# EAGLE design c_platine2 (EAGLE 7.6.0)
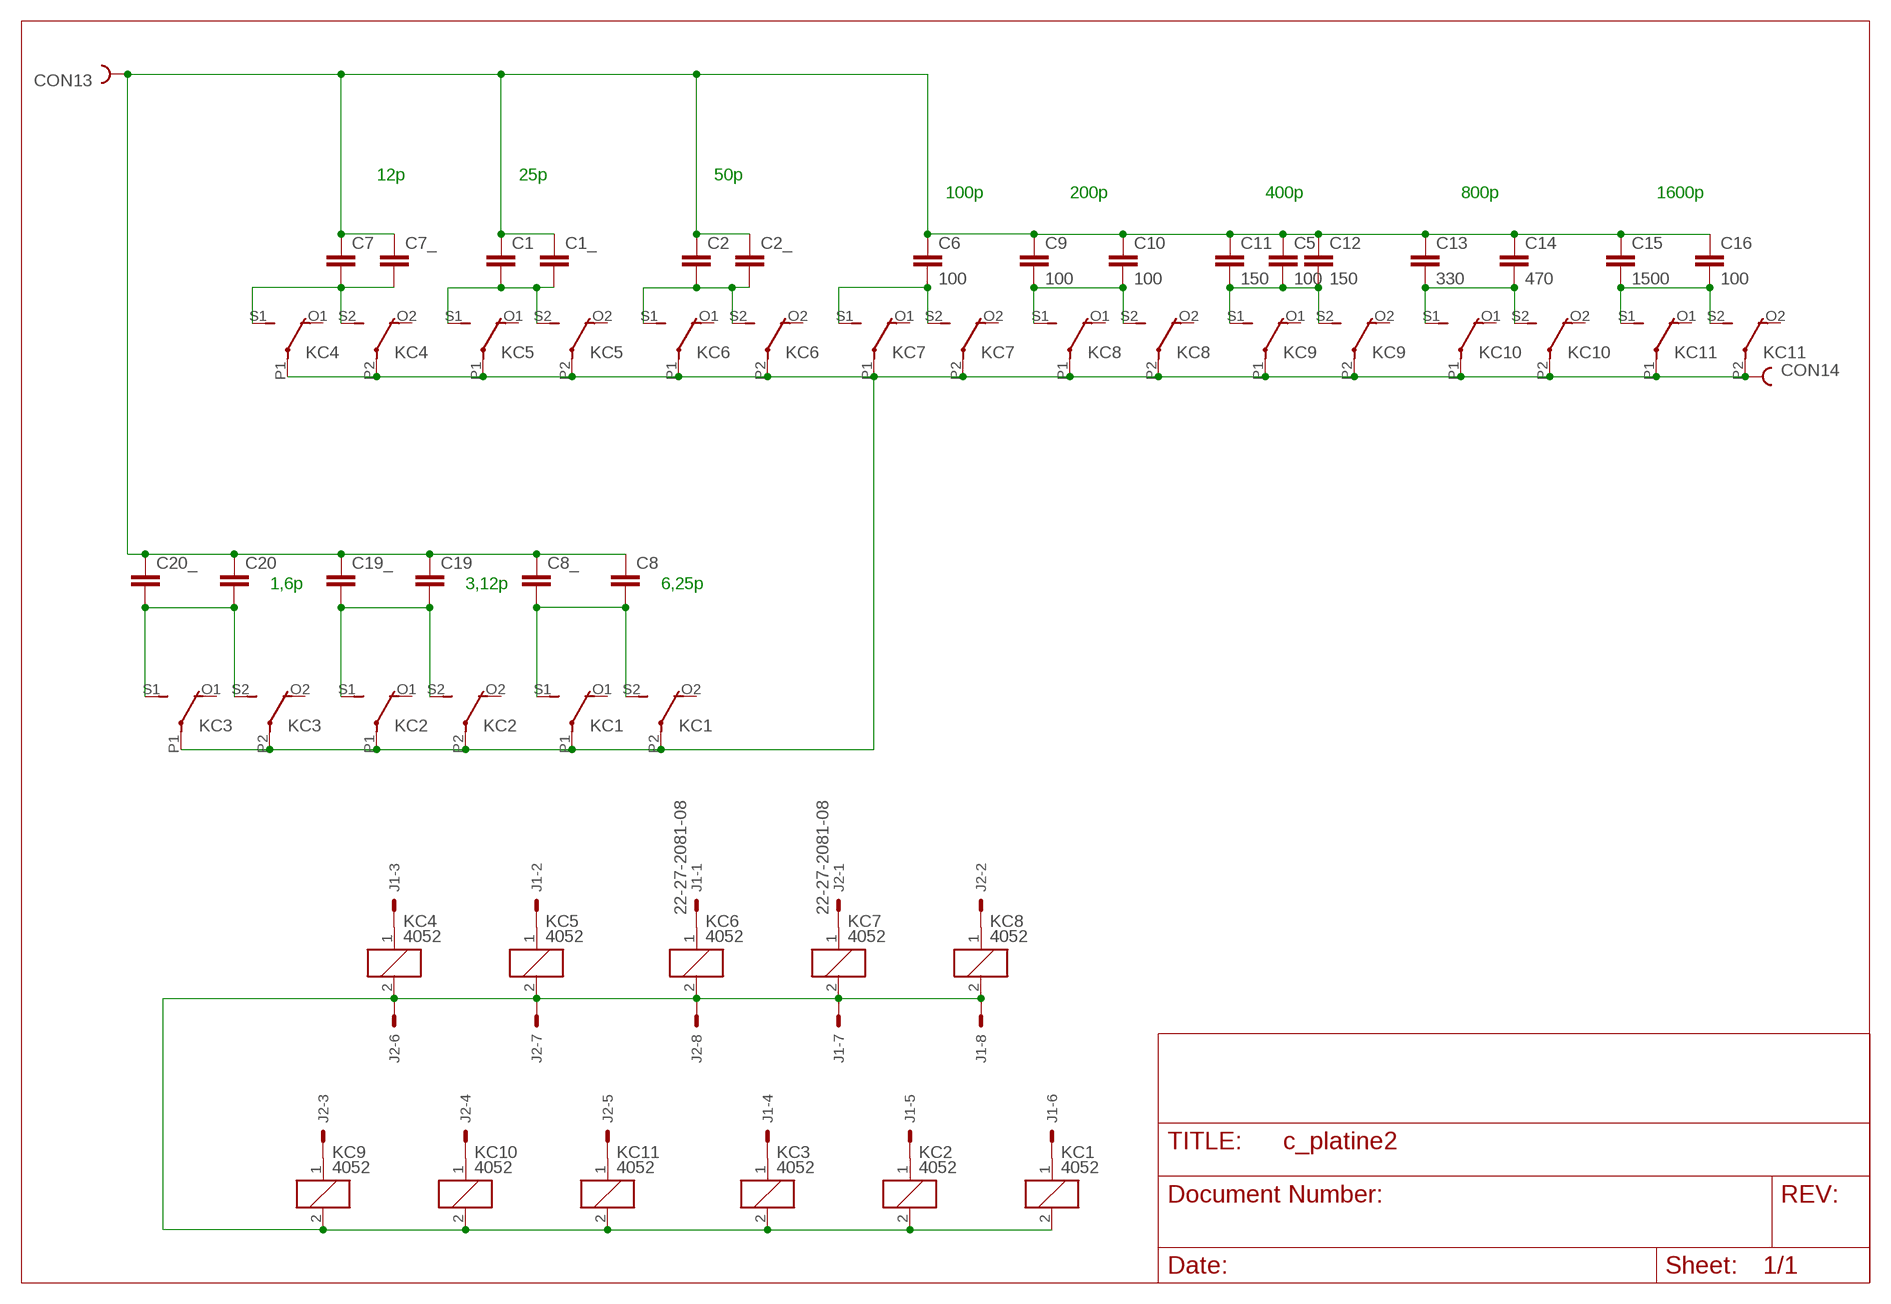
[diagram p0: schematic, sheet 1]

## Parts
C1  C-EUC1812K  [C1812K]
C1_  C-EU102-043X133  [C102-043X133]
C2  C-EUC1812K  [C1812K]
C2_  C-EU102-043X133  [C102-043X133]
C5  100  C-EU150-054X183  [C150-054X183]
C6  100  C-EU150-054X183  [C150-054X183]
C7  C-EUC1812K  [C1812K]
C7_  C-EU102-043X133  [C102-043X133]
C8  C-EUC1812K  [C1812K]
C8_  C-EU102-043X133  [C102-043X133]
C9  100  C-EU150-054X183  [C150-054X183]
C10  100  C-EU150-054X183  [C150-054X183]
C11  150  C-EU150-054X183  [C150-054X183]
C12  150  C-EU150-054X183  [C150-054X183]
C13  330  C-EU150-054X183  [C150-054X183]
C14  470  C-EU150-054X183  [C150-054X183]
C15  1500  C-EU225-074X268  [C225-074X268]
C16  100  C-EU150-054X183  [C150-054X183]
C19  C-EUC1812K  [C1812K]
C19_  C-EU102-043X133  [C102-043X133]
C20  C-EUC1812K  [C1812K]
C20_  C-EU102-043X133  [C102-043X133]
CON13  PIN2_53MM  [HOLE3]
CON14  PIN2_53MM  [HOLE3]
J1  22-27-2081-08  [6410-08]
J2  22-27-2081-08  [6410-08]
KC1  4052  [F4052]
KC2  4052  [F4052]
KC3  4052  [F4052]
KC4  4052  [F4052]
KC5  4052  [F4052]
KC6  4052  [F4052]
KC7  4052  [F4052]
KC8  4052  [F4052]
KC9  4052  [F4052]
KC10  4052  [F4052]
KC11  4052  [F4052]

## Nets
N$1: CON14.1 KC1.P1(2:P) KC1.P2(3:P) KC2.P1(2:P) KC2.P2(3:P) KC3.P1(2:P) KC3.P2(3:P) KC4.P1(2:P) KC4.P2(3:P) KC5.P1(2:P) KC5.P2(3:P) KC6.P1(2:P) KC6.P2(3:P) KC7.P1(2:P) KC7.P2(3:P) KC8.P1(2:P) KC8.P2(3:P) KC9.P1(2:P) KC9.P2(3:P) KC10.P1(2:P) KC10.P2(3:P) KC11.P1(2:P) KC11.P2(3:P)
N$2: C8.2 C8_.2 KC1.S1(2:S) KC1.S2(3:S)
N$3: C1.2 C1_.2 KC5.S1(2:S) KC5.S2(3:S)
N$4: C2.2 C2_.2 KC6.S1(2:S) KC6.S2(3:S)
N$5: C6.2 KC7.S1(2:S) KC7.S2(3:S)
N$6: C7.2 C7_.2 KC4.S1(2:S) KC4.S2(3:S)
N$7: C9.2 C10.2 KC8.S1(2:S) KC8.S2(3:S)
N$8: C5.2 C11.2 C12.2 KC9.S1(2:S) KC9.S2(3:S)
N$9: C13.2 C14.2 KC10.S1(2:S) KC10.S2(3:S)
N$10: C15.2 C16.2 KC11.S1(2:S) KC11.S2(3:S)
N$12: J1.6 KC1.1
N$13: J1.5 KC2.1
N$14: J1.2 KC5.1
N$15: C1.1 C1_.1 C2.1 C2_.1 C5.1 C6.1 C7.1 C7_.1 C8.1 C8_.1 C9.1 C10.1 C11.1 C12.1 C13.1 C14.1 C15.1 C16.1 C19.1 C19_.1 C20.1 C20_.1 CON13.1
N$16: J1.7 J1.8 J2.6 J2.7 J2.8 KC1.2 KC2.2 KC3.2 KC4.2 KC5.2 KC6.2 KC7.2 KC8.2 KC9.2 KC10.2 KC11.2
N$17: J1.1 KC6.1
N$18: C20.2 C20_.2 KC3.S1(2:S) KC3.S2(3:S)
N$19: J2.1 KC7.1
N$20: C19.2 C19_.2 KC2.S1(2:S) KC2.S2(3:S)
N$21: J1.4 KC3.1
N$22: J2.5 KC11.1
N$23: J2.3 KC9.1
N$24: J2.4 KC10.1
N$25: J2.2 KC8.1
N$26: J1.3 KC4.1
Unconnected: KC1.O1(2:O) KC1.O2(3:O) KC2.O1(2:O) KC2.O2(3:O) KC3.O1(2:O) KC3.O2(3:O) KC4.O1(2:O) KC4.O2(3:O) KC5.O1(2:O) KC5.O2(3:O) KC6.O1(2:O) KC6.O2(3:O) KC7.O1(2:O) KC7.O2(3:O) KC8.O1(2:O) KC8.O2(3:O) KC9.O1(2:O) KC9.O2(3:O) KC10.O1(2:O) KC10.O2(3:O) KC11.O1(2:O) KC11.O2(3:O)

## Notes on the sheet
- 12p | 25p | 50p
- 100p | 200p | 400p | 800p | 1600p
- 1,6p | 3,12p | 6,25p

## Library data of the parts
C1 C1_ C2 C2_ C5-C7 C7_ C8 C8_ C9-C16 C19 C19_ C20 C20_ = rcl:C-EU: CAPACITOR, European symbol
CON13 CON14 = lindenau:PIN2_5
J1 J2 = con-molex:22-?-08: CONNECTOR wire to board 2.54 mm (.1 inch) pitch header; OC_FARNELL: unknown; OC_NEWARK: unknown
KC1-KC11 = relay:4052: RELAY 2 x switch, Finder; OC_FARNELL: unknown; OC_NEWARK: unknown

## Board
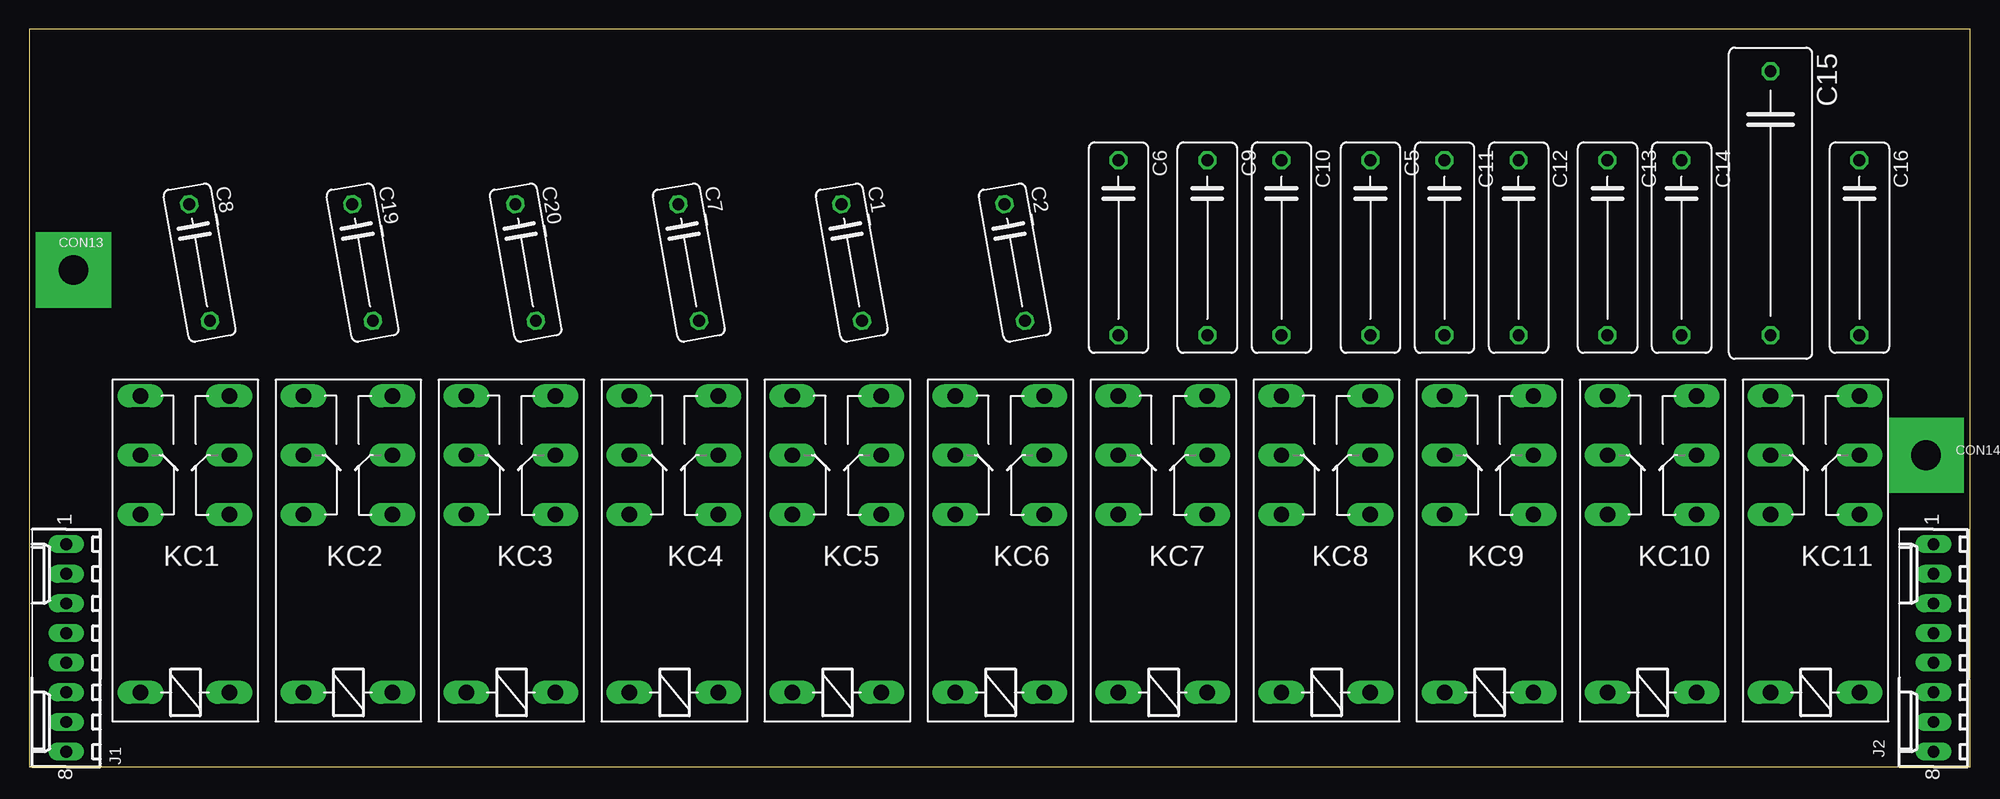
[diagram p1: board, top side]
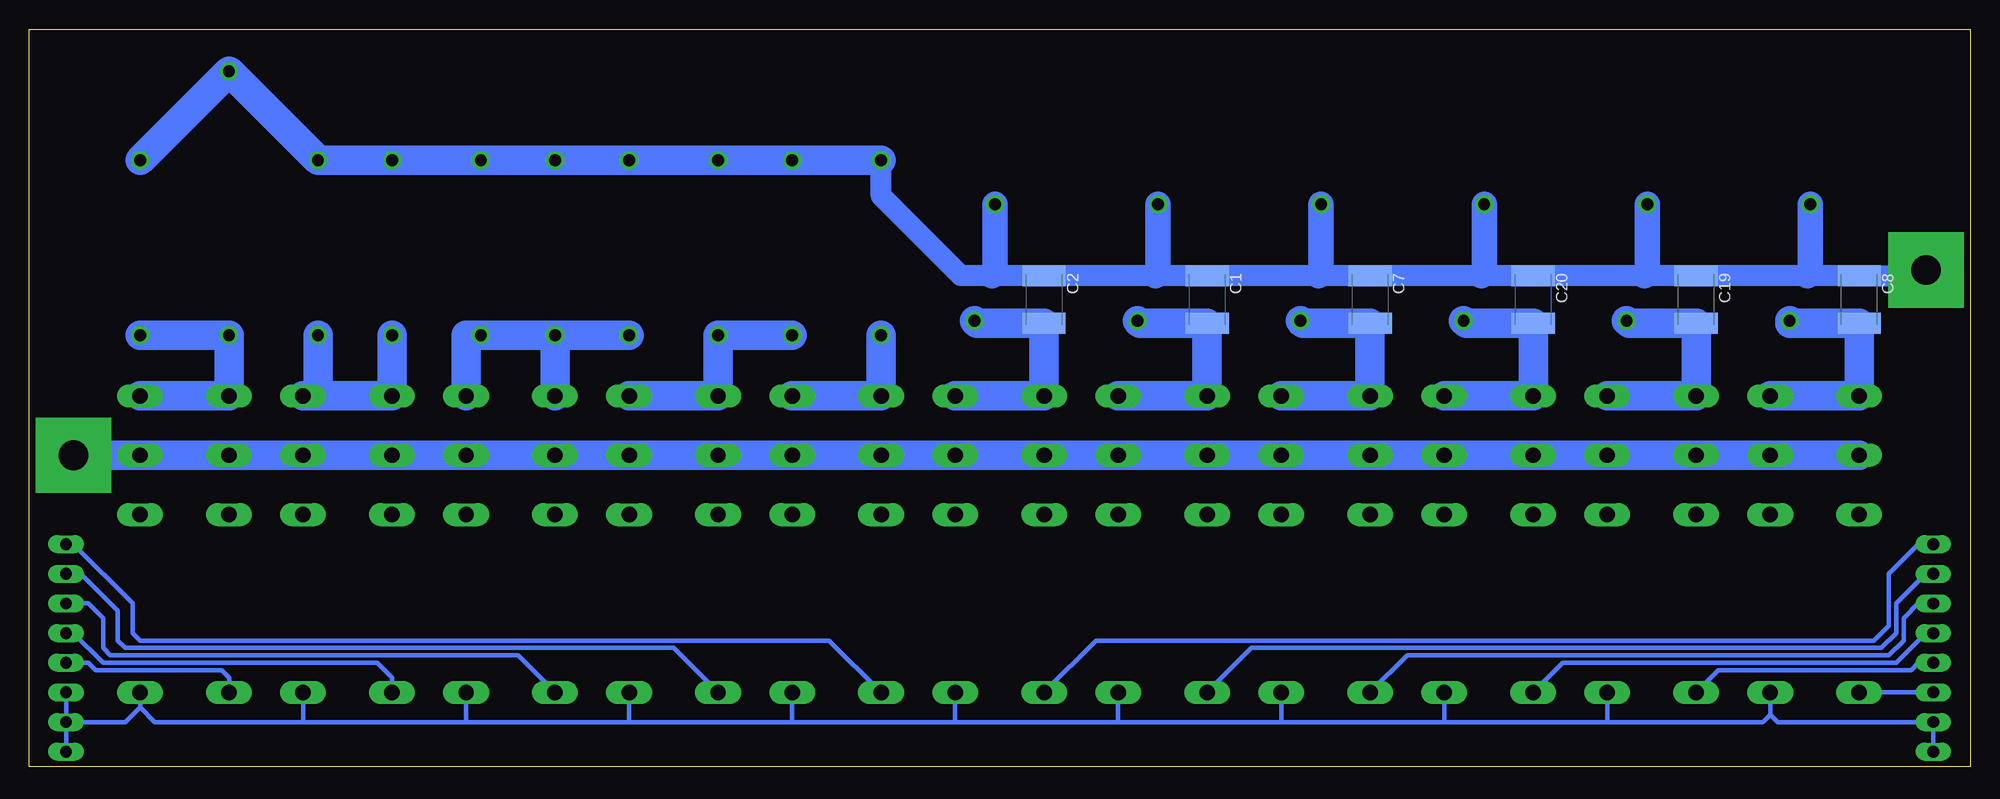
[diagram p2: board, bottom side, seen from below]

Size 166.35 x 63.17 mm. Coordinates in mm from the lower left corner, seen from the top.
Outline: 0,0 166.35,0 166.35,63.17 0,63.17 0,0
Copper layers (1*16): Top 0.035mm / dielectric 1.5mm / Bottom 0.035mm
Design rules "default": minimum track width 10mil, minimum drill 24mil, track to track 8mil, track to pad 8mil, pad to pad 8mil, via to via 8mil, smd to smd 8mil, copper to edge 40mil, drill to drill 8mil, minimum pad ring 10mil, minimum via ring 8mil, stop-mask expansion 4mil, vias tented up to drill 0mil, thermal gap 10mil

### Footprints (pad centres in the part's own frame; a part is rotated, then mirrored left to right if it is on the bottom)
C1812K = smd 1.8 x 3.7: 1 -2.05,0; 2 2.05,0
C102-043X133 = drill 1.016 octagon: 1 -5.08,0; 2 5.08,0
C150-054X183 = drill 1.016 octagon: 1 -7.493,0; 2 7.493,0
C225-074X268 = drill 1.016 octagon: 1 -11.303,0; 2 11.303,0
HOLE3 = drill 2.54 pad 6.452 square: 1 0,0
6410-08 = drill 1.016 long: 1 8.89,0; 2 6.35,0; 3 3.81,0; 4 1.27,0; 5 -1.27,0; 6 -3.81,0; 7 -6.35,0; 8 -8.89,0
F4052 = drill 1.321 long: 1 -3.81,3.81; 2 -3.81,-3.81; O1 11.43,-3.81; O2 11.43,3.81; P1 16.51,-3.81; P2 16.51,3.81; S1 21.59,-3.81; S2 21.59,3.81

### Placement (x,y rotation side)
C1  65.41,40.01 270 bottom
C1_  70.48,43.18 280 top
C2  79.38,40.01 270 bottom
C2_  84.45,43.18 280 top
C5  114.94,44.45 270 top
C6  93.34,44.45 270 top
C7  51.43,40.01 270 bottom
C7_  56.52,43.18 280 top
C8  9.52,40.01 270 bottom
C8_  14.61,43.18 280 top
C9  100.97,44.45 270 top
C10  107.31,44.45 270 top
C11  121.28,44.45 270 top
C12  127.63,44.45 270 top
C13  135.26,44.45 270 top
C14  141.61,44.45 270 top
C15  149.23,48.26 270 top
C16  156.84,44.45 270 top
C19  23.5,40.01 270 bottom
C19_  28.57,43.18 280 top
C20  37.46,40.01 270 bottom
C20_  42.54,43.18 280 top
CON13  3.81,42.55 0 top
CON14  162.56,26.67 0 top
J1  3.17,10.16 90 top
J2  163.2,10.16 90 top
KC1  13.34,10.16 90 top
KC2  27.3,10.16 90 top
KC3  41.27,10.16 90 top
KC4  55.24,10.16 90 top
KC5  69.22,10.16 90 top
KC6  83.19,10.16 90 top
KC7  97.16,10.16 90 top
KC8  111.12,10.16 90 top
KC9  125.09,10.16 90 top
KC10  139.06,10.16 90 top
KC11  153.04,10.16 90 top

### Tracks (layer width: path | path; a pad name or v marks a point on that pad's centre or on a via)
N$1
  Bottom 2.54: KC1.P1 KC1.P2 KC2.P2 KC2.P1 KC3.P2 | KC3.P2 38.73,26.67 | KC3.P2 KC3.P1 KC4.P2 KC4.P1 KC5.P2 KC5.P1 KC6.P2 KC6.P1 KC7.P2 KC7.P1 KC8.P2 KC8.P1 KC9.P2 KC9.P1 KC10.P2 KC10.P1 KC11.P2 KC11.P1 CON14.1
N$2
  Bottom 2.54: 14.61,31.75 KC1.S2 C8.2 15.49,37.95 C8_.2 | 14.61,31.75 KC1.S1 | 14.64,31.78 14.61,31.75
N$3
  Bottom 2.54: 70.48,31.75 KC5.S2 C1.2 71.14,37.95 C1_.2 | 70.48,31.75 KC5.S1 | 70.52,31.78 70.48,31.75
N$4
  Bottom 2.54: 84.45,31.75 KC6.S2 C2.2 85.11,37.95 C2_.2 | 84.45,31.75 KC6.S1 | 84.49,31.78 84.45,31.75
N$5
  Bottom 2.54: C6.2 KC7.S2 KC7.S1
N$6
  Bottom 2.54: 56.52,31.75 KC4.S2 C7.2 57.17,37.95 C7_.2 | 56.52,31.75 KC4.S1 | 56.55,31.78 56.52,31.75
N$7
  Bottom 2.54: C9.2 C10.2 KC8.S2 KC8.S1
N$8
  Bottom 2.54: C5.2 C11.2 | C11.2 C12.2 128.91,36.96 KC9.S1 | C11.2 KC9.S2
N$9
  Bottom 2.54: 141.61,31.75 KC10.S2 C13.2 | 141.61,31.75 KC10.S1 | 141.61,31.75 C14.2
N$10
  Bottom 2.54: KC11.S1 KC11.S2 C15.2 C16.2
N$12
  Bottom 0.406: J1.6 KC1.1
N$13
  Bottom 0.406: J1.5 4.45,8.89 5.08,8.26 21.59,8.26 KC2.1
N$14
  Bottom 0.406: KC5.1 61.59,10.16 7.62,10.16 6.35,11.43 6.35,13.97 3.81,16.51 J1.2
N$15
  Bottom 1.778: C6.1 93.34,48.9 86.5,42.05 83.82,42.05 C2.1 69.85,42.05 C1.1 55.88,42.05 C7.1 41.91,42.05 C20.1 27.94,42.05 C19.1 13.97,42.05 C8.1 4.3,42.05 CON13.1
  Bottom 2.184: C8_.1 13.72,42.3 13.97,42.05 | C19_.1 27.69,42.3 27.94,42.05 | C20_.1 41.66,42.3 41.91,42.05 | C7_.1 55.63,42.3 55.88,42.05 | C1_.1 69.6,42.3 69.85,42.05 | C2_.1 83.57,42.3 83.82,42.05
  Bottom 2.54: C16.1 C15.1 C14.1 C13.1 C12.1 C11.1 C5.1 C10.1 C9.1 C6.1
N$16
  Bottom 0.406: KC1.2 17.14,4.45 | 17.14,4.45 17.78,3.81 31.12,3.81 | 31.12,3.81 45.08,3.81 | 45.08,3.81 59.05,3.81 | 59.05,3.81 73.02,3.81 | 73.02,3.81 86.99,3.81 | 86.99,3.81 100.97,3.81 | 100.97,3.81 114.94,3.81 | 114.94,3.81 128.91,3.81 | 128.91,3.81 142.88,3.81 | 142.88,3.81 155.58,3.81 156.84,5.08 | 156.84,5.08 KC11.2 | KC10.2 142.88,3.81 | KC9.2 128.91,3.81 | KC8.2 114.94,3.81 | KC7.2 100.97,3.81 | KC6.2 86.99,3.81 | KC5.2 73.02,3.81 | KC4.2 59.05,3.81 | KC3.2 45.08,3.81 | KC2.2 31.12,3.81 | J1.8 J1.7 16.51,3.81 17.14,4.45 | J2.8 J2.7 | J2.7 158.12,3.81 156.84,5.08 | J2.7 J2.6
N$17
  Bottom 0.406: KC6.1 74.93,10.79 8.25,10.79 6.98,12.06 6.98,16.51 4.45,19.05 J1.1
N$18
  Bottom 2.54: 42.54,31.75 KC3.S2 C20.2 43.2,37.95 C20_.2 | 42.54,31.75 KC3.S1 | 42.58,31.78 42.54,31.75
N$19
  Bottom 0.406: J2.1 162.56,19.05 157.48,13.97 157.48,11.43 156.84,10.79 97.79,10.79 KC7.1
N$20
  Bottom 2.54: 28.57,31.75 KC2.S2 C19.2 29.23,37.95 C19_.2 | 28.57,31.75 KC2.S1 | 28.61,31.78 28.57,31.75
N$21
  Bottom 0.406: J1.4 3.81,11.43 6.35,8.89 34.92,8.89 KC3.1
N$22
  Bottom 0.406: J2.5 161.29,8.89 160.66,8.26 149.86,8.26 149.23,7.62 KC11.1
N$23
  Bottom 0.406: J2.3 161.29,13.97 160.02,12.7 160.02,10.16 159.39,9.53 124.46,9.53 KC9.1
N$24
  Bottom 0.406: J2.4 162.56,11.43 160.02,8.89 136.53,8.89 135.26,7.62 KC10.1
N$25
  Bottom 0.406: J2.2 161.93,16.51 158.75,13.34 158.75,10.79 158.12,10.16 111.12,10.16 KC8.1
N$26
  Bottom 0.406: KC4.1 48.26,9.53 6.98,9.53 5.71,10.79 5.71,12.7 4.45,13.97 J1.3

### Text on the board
tDocu: 1600p | 1,6p | 3,12p | 6,3p | 12,5p | 25p | 50p | 100p | 200p | 400p | 800p | KC6 | KC7 | KC5 | KC8 | KC4 | KC9 | KC3 | KC10 | KC2 | KC11 | KC1 | 12V | 12V | 12V | 12V | 12V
